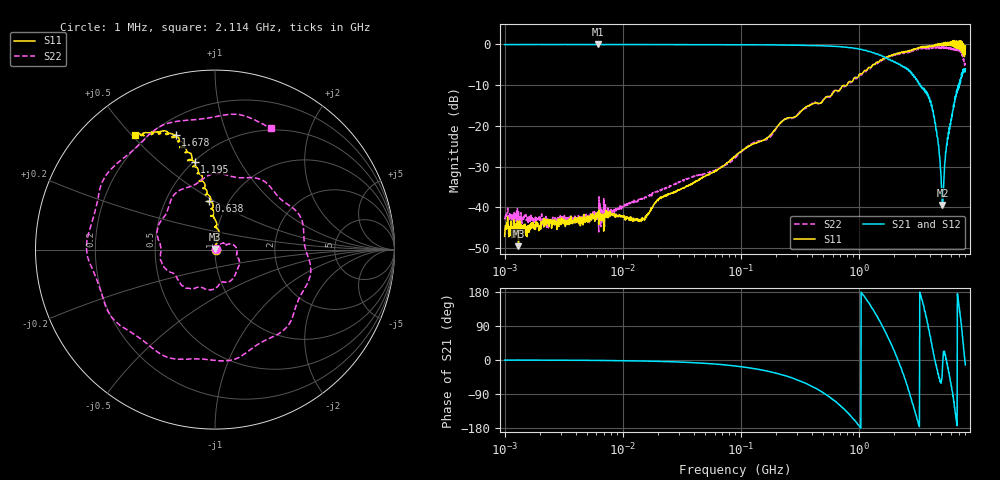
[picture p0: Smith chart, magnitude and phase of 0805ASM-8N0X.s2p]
!s-Parameter Generated by FASTRON Sdn. Bhd.
!FASTRON P/N : 0805ASM-8N0X
!Keysight Technologies: E5071C_MY46733604_B.14.02
!Date: Fri Jun 19 14:46:58 2026
!Version  :Rev00  Fri Jun 19 14:46:58 2026
!Data & Calibration Information:
!Freq  S11:SOLT2(ON)  S21:SOLT2(ON)  S12:SOLT2(ON)  S22:SOLT2(ON)
!PortZ  Port1:50+j0  Port2:50+j0
!When reading reference impedance value at option line is always used.
! Remarks : This data is being provided solely for informational purposes.
# Hz S dB R 50
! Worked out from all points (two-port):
!   1601 points, 1 MHz to 8 GHz, reference 50 ohm
!   highest |S21| = -0.05 dB at 6.17 MHz (marker M1); lowest = -39.4 dB at 5.108 GHz (marker M2)
!   |S21| within 3 dB of the highest: start of sweep to 1.645 GHz
!   lowest |S11| = -49.5 dB at 1.31 MHz (marker M3), VSWR 1.01, Z = 50.2 + j0.287 ohm
!   |S11| at or under -10 dB: start of sweep to 792.5 MHz
!   |S22| runs from -46.0 to -0.6 dB; largest |S21 - S12| = 0.016
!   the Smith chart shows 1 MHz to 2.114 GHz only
!   S11 on the Smith chart (normalised r, x): 1 MHz: 1.01, +0.00; 638 MHz: 0.81, +0.47; 1.195 GHz: 0.50, +0.66; 1.678 GHz: 0.29, +0.67; 2.114 GHz: 0.16, +0.51
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1000000  -47.10 2.4  -0.09 -0.2  -0.06 -0.2  -42.60 4.4
1310238  -49.50 58.6  -0.12 -0.0  -0.07 -0.3  -40.80 -12.6
4479405  -43.40 19.3  -0.08 -0.8  -0.07 -0.9  -42.90 21.3
6169754  -41.10 32.2  -0.05 -1.2  -0.04 -1.1  -41.50 25.0
2.00676e7  -38.00 59.6  -0.08 -3.6  -0.08 -3.5  -36.00 46.8
8.994653e7  -27.40 74.0  -0.11 -15.9  -0.11 -15.8  -27.80 46.1
4.006501e8  -14.70 92.8  -0.33 -69.3  -0.32 -69.2  -14.50 -56.2
6.379863e8  -11.30 97.3  -0.55 -110.0  -0.55 -110.0  -11.40 -138.0
1.19487e9  -5.96 103.0  -1.74 154.0  -1.74 154.0  -5.88 22.4
1.677723e9  -3.42 109.0  -3.36 73.9  -3.34 73.7  -3.28 -145.0
1.7949e9  -2.86 113.0  -3.79 56.0  -3.78 55.8  -2.91 176.0
2.114474e9  -2.17 125.0  -4.58 5.5  -4.58 5.4  -2.57 65.2
2.560258e9  -1.90 136.0  -6.18 -66.0  -6.19 -66.0  -1.83 -90.8
3.044443e9  -1.19 143.0  -8.64 -144.0  -8.63 -144.0  -1.16 105.0
3.345355e9  -0.87 157.0  -10.40 172.0  -10.30 172.0  -0.93 3.2
3.60885e9  -0.66 165.0  -11.30 129.0  -11.30 129.0  -0.88 -90.5
4.095302e9  -0.52 167.0  -14.60 48.3  -14.60 47.6  -0.79 100.0
4.660546e9  0.07 -166.0  -22.90 -32.8  -23.00 -33.0  -0.81 -97.8
5.108415e9  -0.28 -141.0  -39.40 -25.5  -39.50 -25.9  -0.91 118.0
5.696244e9  -0.06 -132.0  -23.10 -21.0  -23.10 -20.7  -0.97 -73.3
6.265031e9  -0.46 -94.3  -16.20 -95.8  -16.20 -95.9  -1.04 98.4
8e9  -0.51 -48.9  -6.03 -12.8  -5.83 -12.5  -5.18 -125.0
